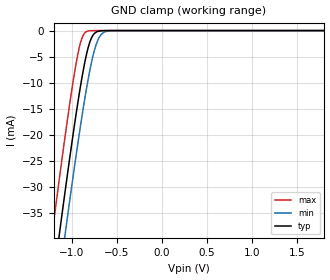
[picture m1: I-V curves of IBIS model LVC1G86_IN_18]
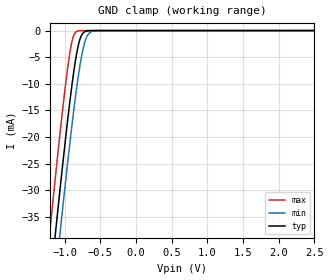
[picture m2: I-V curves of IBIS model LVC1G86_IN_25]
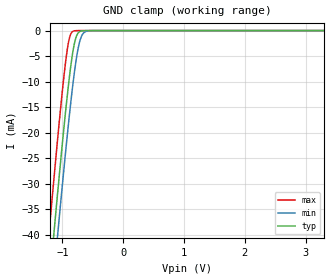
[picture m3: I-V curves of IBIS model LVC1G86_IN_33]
| TEXAS INSTRUMENTS INCORPORATED
| Standard Linear and Logic Group
| IBIS Model of SN74LVC1G86
| SINGLE 2-INPUT EXCLUSIVE-OR GATE
| This file contains package information for the following:
|  SOT 5-pin (DBV) package as [Component] LVC1G86_DBV
|  SOT 5-pin (DCK) package as [Component] LVC1G86_DCK
|  NanoStar WCSP 5-pin (YEA) package as [Component] LVC1G86_YEA
|  NanoFree WCSP 5-pin (YZA) package as [Component] LVC1G86_YZA
| This device can be powered at the following Vccs:
|  1.8 volt Vcc
|  2.5 volt Vcc
|  3.3 volt Vcc
|  5 volt Vcc
| This file provides unique models under the [Model Selector] for each Vcc.
| For operation at a specific Vcc, select the appropriate model after each
| [Model Selector] keyword.
[IBIS Ver]   3.2
[Comment char]  |_char
[File Name]   sn74lvc1g86.ibs
[File Rev]   1.1 | d_die
[Date]   July 24, 2002
[Source]   Data created from TI-SPICE simulations at TI-SLL.
[Notes]   The following is an IBIS list for the LVC1G86D.
   Please contact sllibis@ti.com with questions and
   comments concerning SLL IBIS models.
   - Power-clamp data has been deleted since there is no
   power-clamp diode in the device.
   - C_comp values are taken at a different test condition than
   the Ci in data sheet.
   -Due to the fact that the Device is 5.5-V Input tolarent,
   the pulldown model has some Non-Monotonic Warnings.
[Disclaimer] Property of Texas Instruments Incorporated.  Unauthorized
   reproduction and/or distribution is strictly prohibited.
   This product is protected under copyright law.
   Created  2002, (C) Copyright  2002, Texas Instruments
   Incorporated, All Rights Reserved
   UNLESS THERE IS A SIGNED, WRITTEN AGREEMENT TO THE
   CONTRARY, TEXAS INSTRUMENTS (TI) IS PROVIDING THE IBIS
   MODELS  AND WITHOUT ANY WARRANTY, EXPRESSED OR
   IMPLIED.  TI assumes no liability for:
   1) the accuracy of the IBIS models provided to your
   company;
   2) the proper functioning of these IBIS Models in your
   design or for any resulting applications; or
   3) infringement of patents, copyrights or intellectual
   property rights resulting from your use of these IBIS
   models.
   TI provides IBIS Models as a service to our customers.
   You and your company shall not distribute, sell or give
   these models to anyone else without prior written
   permission from TI.
   TI reserves the right to make changes to our products or
   to discontinue any semiconductor product or service
   without notice, and advises our customers to obtain the
   latest version of relevant information to verify, before
   placing orders, that the information being relied on is
   current.
   Please be aware that your receipt and use of the IBIS
   information provided shall serve as acceptance of these
   terms and conditions.  If you do not accept these terms,
   you should return or destroy the IBIS models and any
   other accompanying information immediately.
| Component LVC1G86_DBV 5-pin SOT
[Component]   LVC1G86_DBV
[Manufacturer]   Texas Instruments, Inc.
[Package]
|   typ   min   max
R_pkg   2.500e-02   2.100e-02   2.900e-02
L_pkg   1.529e-09   1.312e-09   1.906e-09
C_pkg   1.560e-13   1.100e-13   2.400e-13
[Pin]   signal_name   model_name   R_pin   L_pin   C_pin
1   A   LVC1G86_IN   2.100e-02   1.511e-09   1.440e-13
2   B   LVC1G86_IN   2.300e-02   1.312e-09   1.380e-13
3   GND   GND   2.900e-02   1.906e-09   2.400e-13
4   Y   LVC1G86_OUT   2.600e-02   1.541e-09   1.500e-13
5   VCC   POWER   2.500e-02   1.374e-09   1.100e-13
| Component LVC1G86_DCK 5-pin SOT
[Component]   LVC1G86_DCK
[Manufacturer]   Texas Instruments, Inc.
[Package]
|   typ   min   max
R_pkg   2.000e-02   1.700e-02   2.500e-02
L_pkg   9.980e-10   8.810e-10   1.069e-09
C_pkg   1.460e-13   1.180e-13   2.050e-13
[Pin]   signal_name   model_name   R_pin   L_pin   C_pin
1   A   LVC1G86_IN   1.900e-02   1.069e-09   1.620e-13
2   B   LVC1G86_IN   1.800e-02   8.810e-10   1.210e-13
3   GND   GND   1.700e-02   1.031e-09   2.050e-13
4   Y   LVC1G86_OUT   2.000e-02   9.600e-10   1.240e-13
5   VCC   POWER   2.500e-02   1.049e-09   1.180e-13
| Component LVC1G86_YEA 5-pin NanoStar WCSP
[Component]   LVC1G86_YEA
[Manufacturer]   Texas Instruments, Inc.
[Package]
|   typ   min   max
R_pkg   0.001   0.001   0.001
L_pkg   0.021nH   0.021nH   0.021nH
C_pkg   0.046pF   0.045pF   0.047pF
[Pin]   signal_name   model_name   R_pin   L_pin   C_pin
1   A   LVC1G86_IN   0.001   0.021nH   0.046pF
2   B   LVC1G86_IN   0.001   0.021nH   0.047pF
3   GND   GND   0.001   0.021nH   0.046pF
4   Y   LVC1G86_OUT   0.001   0.021nH   0.045pF
5   VCC   POWER   0.001   0.021nH   0.045pF
| Component LVC1G86_YZA 5-pin NanoFree WCSP
[Component]   LVC1G86_YZA
[Manufacturer]   Texas Instruments, Inc.
[Package]
|   typ   min   max
R_pkg   0.001   0.001   0.001
L_pkg   0.021nH   0.021nH   0.021nH
C_pkg   0.046pF   0.045pF   0.047pF
[Pin]   signal_name   model_name   R_pin   L_pin   C_pin
1   A   LVC1G86_IN   0.001   0.021nH   0.046pF
2   B   LVC1G86_IN   0.001   0.021nH   0.047pF
3   GND   GND   0.001   0.021nH   0.046pF
4   Y   LVC1G86_OUT   0.001   0.021nH   0.045pF
5   VCC   POWER   0.001   0.021nH   0.045pF
| Model LVC1G86_IN
[Model Selector]   LVC1G86_IN
LVC1G86_IN_18   1.8 volt Vcc
LVC1G86_IN_25   2.5 volt Vcc
LVC1G86_IN_33   3.3 volt Vcc
LVC1G86_IN_50   5 volt Vcc
| Model LVC1G86_OUT
[Model Selector]   LVC1G86_OUT
LVC1G86_OUT_18   1.8 volt Vcc
LVC1G86_OUT_25   2.5 volt Vcc
LVC1G86_OUT_33   3.3 volt Vcc
LVC1G86_OUT_50   5 volt Vcc
| Models and submodels in the file (8): LVC1G86_IN_18 (Input), LVC1G86_IN_25 (Input), LVC1G86_IN_33 (Input), LVC1G86_IN_50 (Input), LVC1G86_OUT_18 (Output), LVC1G86_OUT_25 (Output), LVC1G86_OUT_33 (Output), LVC1G86_OUT_50 (Output)
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[Model]   LVC1G86_IN_18
Model_type  Input
Vinl=0.5775
Vinh=1.2675
| variable   typ   min   max
C_comp   3.46pF   3.07pF   4.19pF
[Temperature Range]   40   100   -40
| Ambient temperature   25   85   -40
[Voltage range]   1.8   1.65   1.95
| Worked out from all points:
|   GND clamp passes 1 mA (typ) near -0.77 V on its own axis
[GND Clamp]
| LVC1G86_IN_18
|   Voltage   I(typ)   I(min)   I(max)
-5V       -583.8mA   -590.8mA   -575.1mA
-1.21V    -48.93mA   -57.22mA   -38.3mA
-1.135V   -39.07mA   -47.36mA   -28.42mA
-1.075V   -31.35mA   -39.6mA    -20.75mA
-1.06V    -29.44mA   -37.69mA   -18.89mA
-960mV    -17.26mA   -25.26mA   -7.377mA
-885mV    -9.098mA   -16.55mA   -1.486mA
-830mV    -4.281mA   -10.75mA   -171.6uA
-780mV    -1.472mA   -6.227mA   -17.15uA
-715mV    -205.4uA   -2.128mA   -808.5nA
-650mV    -22.01uA   -443.9uA   -37.93nA
1.8V      3.326pA    6.142pA    3.026pA
[Model]   LVC1G86_IN_25
Model_type  Input
Vinl=0.7
Vinh=1.7
| variable   typ   min   max
C_comp   3.40pF   2.90pF   4.26pF
[Temperature Range]   40   100   -40
| Ambient temperature   25   85   -40
[Voltage range]   2.5   2.3   2.7
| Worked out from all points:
|   GND clamp passes 1 mA (typ) near -0.77 V on its own axis
[GND Clamp]
| LVC1G86_IN_25
|   Voltage   I(typ)   I(min)   I(max)
-5V       -583.8mA   -590.8mA   -575.1mA
-1.205V   -48.27mA   -56.56mA   -37.63mA
-1.13V    -38.42mA   -46.71mA   -27.77mA
-1.07V    -30.71mA   -38.96mA   -20.13mA
-1.05V    -28.19mA   -36.42mA   -17.65mA
-955mV    -16.68mA   -24.66mA   -6.874mA
-885mV    -9.098mA   -16.55mA   -1.486mA
-830mV    -4.281mA   -10.75mA   -171.6uA
-780mV    -1.472mA   -6.227mA   -17.15uA
-710mV    -173.7uA   -1.918mA   -639nA
-645mV    -18.49uA   -387.7uA   -29.98nA
2.5V      4.713pA    7.577pA    4.389pA
[Model]   LVC1G86_IN_33
Model_type  Input
Vinl=0.8
Vinh=2.0
| variable   typ   min   max
C_comp   3.33pF   2.75pF   4.34pF
[Temperature Range]   40   100   -40
| Ambient temperature   25   85   -40
[Voltage range]   3.3   3   3.6
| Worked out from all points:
|   GND clamp passes 1 mA (typ) near -0.77 V on its own axis
[GND Clamp]
| LVC1G86_IN_33
|   Voltage   I(typ)   I(min)   I(max)
-5V       -583.8mA   -590.8mA   -575.1mA
-1.215V   -49.6mA    -57.88mA   -38.96mA
-1.14V    -39.72mA   -48.01mA   -29.07mA
-1.08V    -31.98mA   -40.25mA   -21.38mA
-1.06V    -29.44mA   -37.69mA   -18.89mA
-925mV    -13.29mA   -21.11mA   -4.122mA
-875mV    -8.124mA   -15.45mA   -1.065mA
-820mV    -3.579mA   -9.774mA   -109.4uA
-770mV    -1.128mA   -5.445mA   -10.73uA
-715mV    -205.4uA   -2.128mA   -808.5nA
-590mV    -2.7uA     -81.86uA   -2.255nA
3.3V      6.304pA    9.258pA    5.93pA
